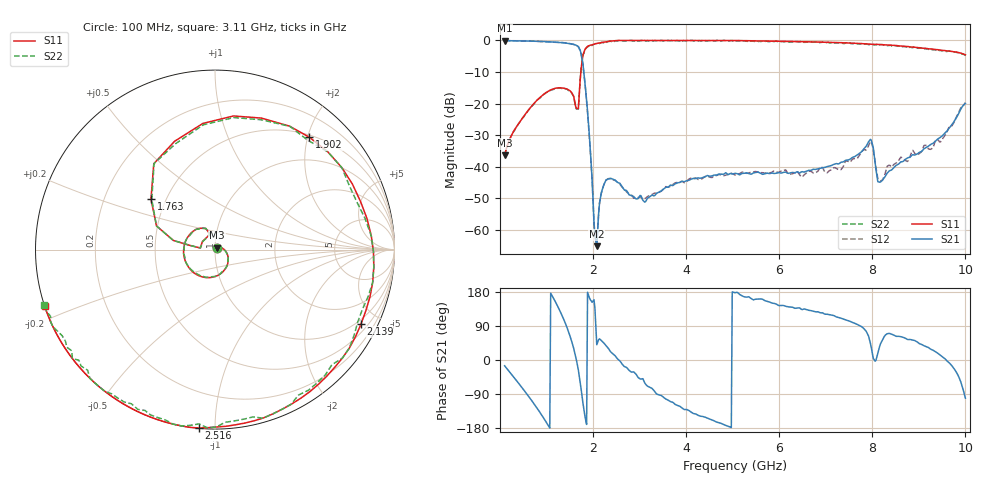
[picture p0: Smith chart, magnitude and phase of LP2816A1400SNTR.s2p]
!	AVX	THIN	FILM	OPERATION
!	LP2816S	High	Performance	Low	Pass	Filters
!	P/N	LP2816A1400SNTR
!	Created	22	November	2016
!Instrument:	"HEWLETT PACKARD,8720ES,US39172150,7.62 "
#	MHz	S	dB	R	50
!	Frq	S11(dB)	S11(deg)	S21(dB)	S21(deg)	S12(dB)	S12(deg)	S22(dB)	S22(deg)
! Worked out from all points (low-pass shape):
!   501 points, 100 MHz to 10 GHz, reference 50 ohm
!   highest |S21| = -0.05 dB at 100 MHz (marker M1); lowest = -65.2 dB at 2.08 GHz (marker M2)
!   |S21| within 3 dB of the highest: start of sweep to 1.722 GHz
!   lowest |S11| = -36.4 dB at 100 MHz (marker M3), VSWR 1.03, Z = 51.1 + j1.05 ohm
!   |S11| at or under -10 dB: start of sweep to 1.738 GHz
!   |S22| runs from -36.4 to 0.0 dB; largest |S21 - S12| = 0.016
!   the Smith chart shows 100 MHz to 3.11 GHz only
!   S11 on the Smith chart (normalised r, x): 100 MHz: 1.02, +0.02; 1.763 GHz: 0.41, +0.29; 1.902 GHz: 0.54, +2.03; 2.139 GHz: 0.81, -4.02; 2.516 GHz: 0.00, -0.91; 3.11 GHz: -0.00, -0.16
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100  -36.43 43.0  -0.05 -15.3  -0.06 -15.3  -36.43 43.0
595  -22.40 -22.9  -0.20 -92.5  -0.17 -92.6  -22.40 -23.0
1010.8  -16.34 -92.6  -0.41 -167.3  -0.44 -167.5  -16.44 -92.7
1228.6  -15.07 -141.3  -0.60 144.6  -0.59 144.3  -15.17 -141.5
1426.6  -15.35 164.3  -0.86 90.2  -0.82 89.6  -15.35 164.2
1624.6  -20.82 108.3  -1.44 10.3  -1.47 9.6  -20.92 108.1
1763.2  -6.85 141.7  -5.78 -95.0  -6.05 -95.2  -6.95 141.6
1901.8  -1.75 49.9  -26.30 171.7  -26.75 173.0  -1.95 49.7
2040.4  -1.08 -0.8  -61.89 136.4  -61.83 154.4  -1.08 -0.8
2080  -0.94 -11.8  -65.22 40.2  -64.96 36.5  -0.94 -11.8
2139.4  -0.79 -26.9  -51.50 56.0  -51.65 49.7  -0.99 -27.1
2515.6  -0.02 -95.1  -44.87 4.5  -44.83 4.0  -0.22 -95.2
3109.6  0.00 -161.8  -51.23 -60.0  -50.16 -59.8  0.00 -161.9
3406.6  0.00 172.8  -48.13 -91.7  -48.25 -87.7  0.00 172.7
4099.6  0.00 125.3  -44.02 -136.8  -43.67 -137.7  0.00 125.1
5050  0.00 75.1  -42.13 177.6  -42.66 177.5  0.00 74.9
6713.2  -0.47 8.4  -40.96 129.4  -41.81 120.1  -0.57 8.3
7940.8  -1.16 -38.6  -31.72 52.8  -32.62 63.4  -1.36 -38.6
8138.8  -1.27 -46.5  -44.85 27.2  -44.14 28.7  -1.27 -46.5
8356.6  -1.45 -56.5  -41.47 70.1  -39.55 65.8  -1.55 -56.5
9227.8  -2.66 -104.2  -33.26 30.9  -34.47 25.6  -2.76 -104.3
10000  -4.54 -165.0  -20.02 -100.8  -19.67 -95.4  -4.74 -165.2
